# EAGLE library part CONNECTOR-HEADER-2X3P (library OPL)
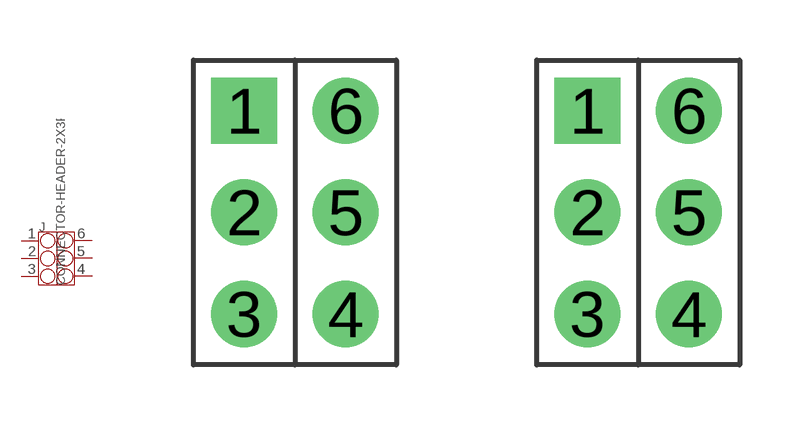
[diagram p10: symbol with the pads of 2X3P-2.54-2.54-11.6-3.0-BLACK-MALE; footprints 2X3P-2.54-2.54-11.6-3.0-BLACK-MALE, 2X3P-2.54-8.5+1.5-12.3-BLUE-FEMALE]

Designator prefix J

## CONNECTOR-HEADER-2X3P-3460180P1  [2X3P-2.54-2.54-11.6-3.0-BLACK-MALE]
1  1
2  2
3  3
4  4
5  5
6  6

## CONNECTOR-HEADER-2X3P-3461240P1  [2X3P-2.54-8.5+1.5-12.3-BLUE-FEMALE]
Pads as for 2X3P-2.54-2.54-11.6-3.0-BLACK-MALE

## Footprint 2X3P-2.54-2.54-11.6-3.0-BLACK-MALE (pad centres in mm)
drill 0.889 pad 1.651 square: 1 -1.27,2.54
drill 0.889 pad 1.651: 2 -1.27,0; 3 -1.27,-2.54; 4 1.27,-2.54; 5 1.27,0; 6 1.27,2.54

## Footprint 2X3P-2.54-8.5+1.5-12.3-BLUE-FEMALE (pad centres in mm)
drill 0.889 pad 1.651 square: 1 -1.27,2.54
drill 0.889 pad 1.651: 2 -1.27,0; 3 -1.27,-2.54; 4 1.27,-2.54; 5 1.27,0; 6 1.27,2.54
